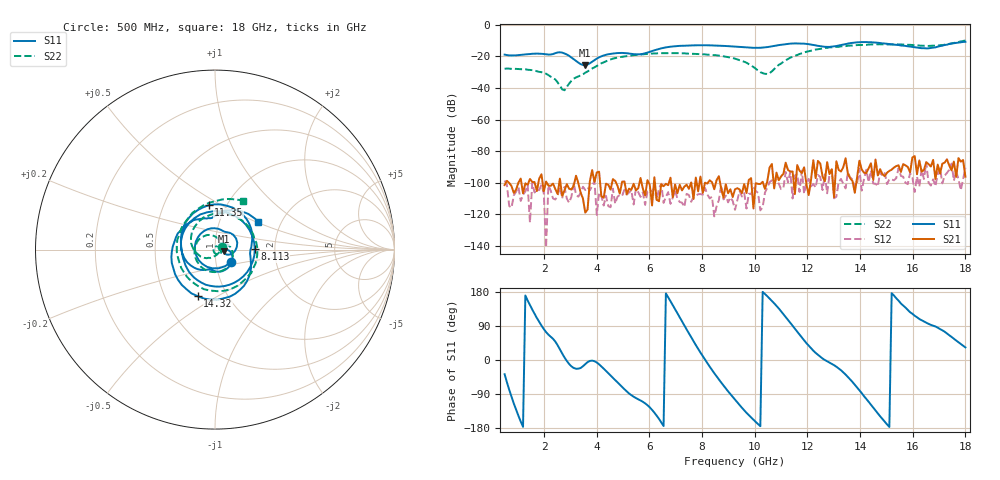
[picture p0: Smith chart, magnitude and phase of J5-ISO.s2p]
!Agilent Technologies,N5230A,MY45001360,A.07.50.67
!Agilent N5230A: A.07.50.67
!Date: Tuesday, April 16, 2024 15:57:30
!Correction: S11(Full 2 Port(1,2))
!S21(Full 2 Port(1,2))
!S12(Full 2 Port(1,2))
!S22(Full 2 Port(1,2))
!S2P File: Measurements: S11, S21, S12, S22:
# Hz S  dB  R 50
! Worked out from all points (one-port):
!   201 points, 500 MHz to 18 GHz, reference 50 ohm
!   lowest |S11| = -25.7 dB at 3.562 GHz (marker M1), VSWR 1.11, Z = 55.3 - j1.11 ohm
!   |S11| at or under -10 dB: start of sweep to end of sweep
!   S11 on the Smith chart (normalised r, x): 500 MHz: 1.18, -0.16; 8.113 GHz: 1.57, +0.01; 11.35 GHz: 0.83, +0.44; 14.32 GHz: 0.73, -0.41; 18 GHz: 1.52, +0.52
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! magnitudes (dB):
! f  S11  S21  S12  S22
! 500 MHz  -19.0  -101.4  -98.6  -27.9
! 1.288 GHz  -18.9  -100.4  -105.5  -28.2
! 2.075 GHz  -18.8  -99.2  -140.9  -31.1
! 2.425 GHz  -18.1  -103.9  -110.6  -34.7
! 2.775 GHz  -18.3  -104.8  -102.6  -41.5
! 3.125 GHz  -22.0  -101.8  -100.1  -34.1
! 3.475 GHz  -25.5  -109.9  -102.5  -31.5
! 3.562 GHz  -25.7  -118.9  -104.6  -30.4
! 4.175 GHz  -20.1  -108.5  -108.3  -24.5
! 4.612 GHz  -18.3  -97.7  -103.6  -21.5
! 5.662 GHz  -18.7  -97.0  -108.9  -18.9
! 6.362 GHz  -15.4  -111.6  -103.7  -18.1
! 8.113 GHz  -13.1  -99.9  -103.3  -18.8
! 9.25 GHz  -13.9  -104.1  -117.1  -21.5
! 10.47 GHz  -14.2  -99.2  -103.2  -31.2
! 11.35 GHz  -12.1  -92.8  -93.1  -20.9
! 12.22 GHz  -12.9  -85.7  -100.8  -16.2
! 12.84 GHz  -14.1  -94.5  -94.9  -14.4
! 14.32 GHz  -11.2  -90.9  -99.6  -12.6
! 15.11 GHz  -12.3  -92.5  -97.8  -12.6
! 16.6 GHz  -15.0  -88.2  -99.9  -13.5
! 18 GHz  -10.9  -96.2  -90.4  -10.0
